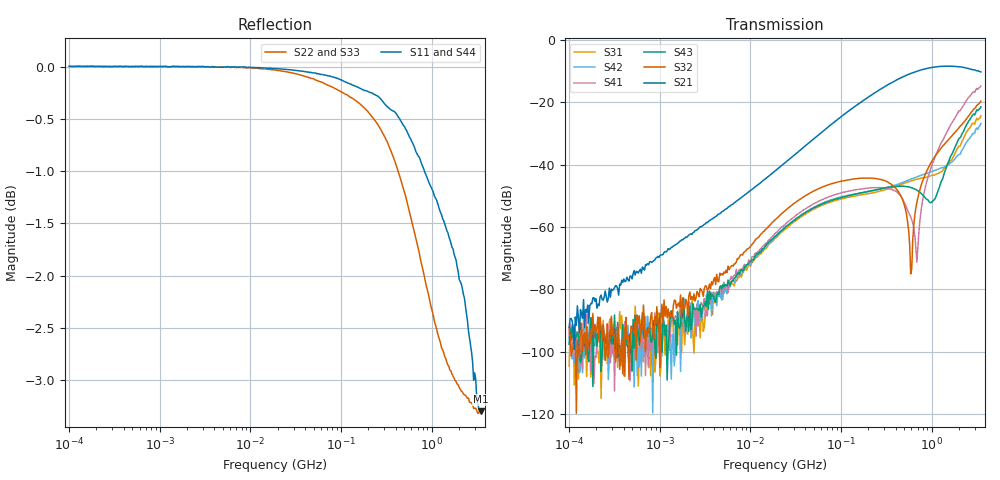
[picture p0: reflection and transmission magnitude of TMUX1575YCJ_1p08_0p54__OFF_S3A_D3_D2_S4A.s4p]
!Keysight Technologies,E5080A,MY55200740,A.12.60.03
!Date: Wednesday, July 22, 2020 12:10:34
!Correction: S11(Full 4 Port(1,2,3,4))
!S12(Full 4 Port(1,2,3,4))
!S13(Full 4 Port(1,2,3,4))
!S14(Full 4 Port(1,2,3,4))
!S21(Full 4 Port(1,2,3,4))
!S22(Full 4 Port(1,2,3,4))
!S23(Full 4 Port(1,2,3,4))
!S24(Full 4 Port(1,2,3,4))
!S31(Full 4 Port(1,2,3,4))
!S32(Full 4 Port(1,2,3,4))
!S33(Full 4 Port(1,2,3,4))
!S34(Full 4 Port(1,2,3,4))
!S41(Full 4 Port(1,2,3,4))
!S42(Full 4 Port(1,2,3,4))
!S43(Full 4 Port(1,2,3,4))
!S44(Full 4 Port(1,2,3,4))
!S4P File: Measurements: <S11,S12,S13,S14>,
!<S21,S22,S23,S24>,
!<S31,S32,S33,S34>,
!<S41,S42,S43,S44>:Log Frequency Sweep
# Hz S  dB  R 50
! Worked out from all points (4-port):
!   400 points, 100 kHz to 3.5 GHz, reference 50 ohm
!   strongest paths, dB at 100 kHz, 1.377 MHz, 18.96 MHz, 261 MHz, 3.5 GHz:
!     S21: -92.1, -66.4, -41.9, -16.2, -10.4
!     S32: -92.4, -88.8, -57.6, -44.6, -19.7
!     S43: -97.6, -88.6, -63.0, -47.9, -21.5
!     S41: -94.4, -86.9, -61.9, -47.4, -14.9
!     S42: -95.4, -94.4, -63.0, -48.1, -26.8
!     S31: -104.6, -86.8, -63.5, -48.6, -24.4
!   lowest |S11| = -3.3 dB at 3.5 GHz (marker M1), VSWR 5.33, Z = 12.1 - j26.1 ohm
!   |S11| at or under -10 dB: nowhere
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100000  0.00 -0.0  -90.60 121.3  -101.95 -45.8  -98.31 -101.5
        -92.13 96.1  0.00 -0.0  -93.86 9.2  -95.99 -147.0
        -104.55 -128.0  -92.38 47.9  0.00 -0.0  -95.95 -124.8
        -94.43 -157.0  -95.43 -37.6  -97.56 74.8  0.00 -0.0
2.172061e8  -0.25 -15.3  -17.72 76.2  -49.18 32.5  -47.47 35.3
            -17.73 76.2  -0.47 -25.3  -44.37 19.3  -48.48 33.1
            -49.14 32.4  -44.38 19.0  -0.48 -26.3  -48.41 33.6
            -47.44 35.2  -48.49 33.1  -48.39 33.5  -0.11 -15.1
4.770142e8  -0.55 -31.3  -12.00 52.7  -46.23 22.4  -50.92 21.8
            -12.00 52.8  -1.14 -50.5  -51.20 -5.5  -45.75 25.7
            -46.21 22.5  -51.18 -5.6  -1.18 -54.3  -46.96 17.5
            -50.91 21.6  -45.75 25.9  -46.95 17.5  -0.53 -32.9
5.883563e8  -0.69 -37.5  -10.85 45.0  -45.28 14.5  -56.76 40.2
            -10.85 45.0  -1.44 -59.6  -75.24 0.0  -44.71 20.9
            -45.29 14.5  -75.04 -3.6  -1.44 -63.5  -47.31 8.9
            -56.79 39.9  -44.71 20.9  -47.33 8.9  -0.64 -39.4
6.886083e8  -0.83 -42.7  -10.13 38.9  -44.69 6.2  -70.69 119.0
            -10.12 38.9  -1.69 -66.7  -52.10 159.9  -43.96 15.6
            -44.68 6.4  -52.07 159.6  -1.70 -71.2  -48.22 -0.2
            -71.25 113.5  -43.94 15.6  -48.20 -0.3  -0.70 -44.6
1.020474e9  -1.18 -57.8  -8.90 23.1  -43.40 -28.6  -39.79 -170.3
            -8.89 23.1  -2.34 -85.2  -38.66 146.4  -42.20 -7.0
            -43.38 -28.6  -38.67 146.3  -2.28 -89.9  -51.85 -71.0
            -39.80 -170.2  -42.19 -7.0  -51.87 -71.1  -1.09 -60.0
3.5e9  -3.30 -122.6  -10.37 -20.5  -24.34 152.0  -14.86 129.0
       -10.36 -20.6  -3.27 -132.7  -19.72 134.4  -26.86 172.2
       -24.37 151.7  -19.73 134.2  -3.69 -144.5  -21.55 135.3
       -14.89 128.8  -26.84 171.7  -21.53 135.2  -3.17 -121.6
